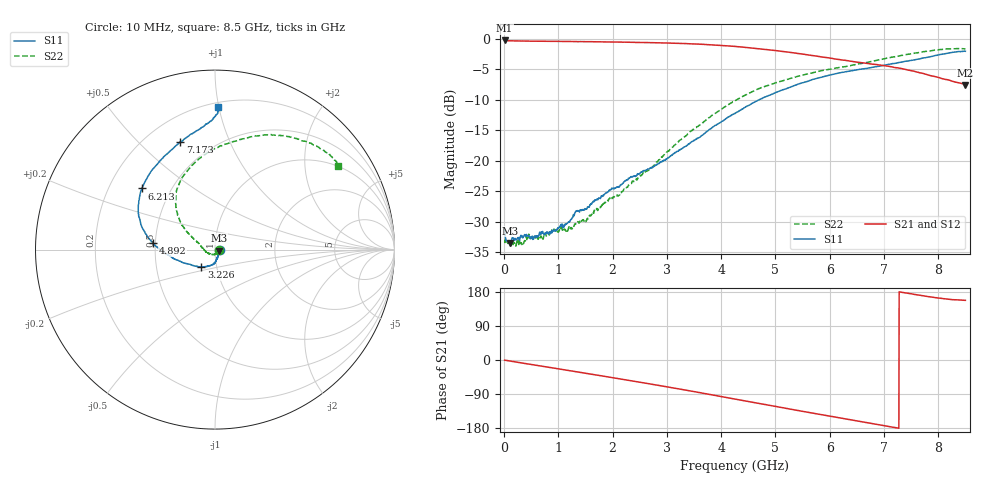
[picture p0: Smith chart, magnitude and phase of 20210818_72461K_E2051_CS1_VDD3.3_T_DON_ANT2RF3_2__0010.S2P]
!Agilent Technologies,E5071C,MY46417908,A.11.23
!Date: Wed Aug 18 14:29:43 2021
!Data & Calibration Information:
!Freq	S11:SOLT2(ON)	S21:SOLT2(ON)	S12:SOLT2(ON)	S22:SOLT2(ON)
!PortZ  Port1:50+j0  Port2:50+j0
!Above PortZ is port z conversion or system Z0 setting when saving the data.
!When reading, reference impedance value at option line is always used.
# Hz S dB R 50
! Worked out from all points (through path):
!   1601 points, 10 MHz to 8.5 GHz, reference 50 ohm
!   highest |S21| = -0.24 dB at 10 MHz (marker M1); lowest = -7.5 dB at 8.5 GHz (marker M2)
!   group delay of S21, straight-line fit = 69 ps
!   lowest |S11| = -33.5 dB at 110.8 MHz (marker M3), VSWR 1.04, Z = 52.1 - j0.533 ohm
!   |S11| at or under -10 dB: start of sweep to 4.69 GHz
!   |S22| runs from -34.0 to -1.6 dB; largest |S21 - S12| = 0.0047
!   S11 on the Smith chart (normalised r, x): 10 MHz: 1.05, +0.00; 3.226 GHz: 0.84, -0.17; 4.892 GHz: 0.49, +0.04; 6.213 GHz: 0.34, +0.32; 7.173 GHz: 0.34, +0.67; 8.5 GHz: 0.23, +1.00
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1e7  -31.69 0.7  -0.24 -0.4  -0.24 -0.4  -33.22 -8.8
1.108188e8  -33.48 -14.0  -0.29 -2.8  -0.29 -2.8  -33.65 -18.7
3.28375e8  -32.30 -25.3  -0.33 -7.8  -0.32 -7.8  -33.66 -45.1
4.451125e8  -32.23 -35.5  -0.34 -10.6  -0.33 -10.6  -32.46 -49.6
6.838938e8  -31.92 -44.8  -0.37 -16.0  -0.36 -16.0  -32.41 -62.0
8.483875e8  -31.86 -54.9  -0.39 -19.8  -0.39 -19.8  -32.00 -74.9
1.177375e9  -30.14 -59.7  -0.41 -27.4  -0.41 -27.4  -31.35 -95.8
1.320644e9  -28.33 -65.4  -0.42 -30.7  -0.42 -30.7  -30.27 -114.2
1.426769e9  -28.16 -67.3  -0.43 -33.2  -0.43 -33.2  -29.72 -125.1
1.516975e9  -27.90 -68.5  -0.44 -35.3  -0.44 -35.3  -29.76 -130.0
2.185562e9  -23.72 -86.7  -0.52 -51.1  -0.52 -51.1  -24.93 -173.9
2.843538e9  -20.41 -108.7  -0.62 -67.0  -0.63 -67.0  -19.93 158.3
3.225588e9  -18.21 -128.2  -0.72 -76.4  -0.72 -76.4  -16.71 151.8
3.692538e9  -15.51 -151.6  -0.88 -88.4  -0.88 -88.4  -13.50 144.7
4.255e9  -12.21 -170.1  -1.22 -103.0  -1.21 -103.0  -10.15 133.6
4.89175e9  -9.22 174.2  -1.79 -119.6  -1.79 -119.6  -7.52 118.0
5.671769e9  -6.69 156.3  -2.70 -139.8  -2.72 -140.0  -5.55 97.0
6.213006e9  -5.49 140.1  -3.41 -153.3  -3.41 -153.5  -4.61 85.2
7.088538e9  -4.16 110.4  -4.49 -175.6  -4.49 -175.7  -3.09 65.8
7.173438e9  -4.03 108.0  -4.64 -177.6  -4.63 -177.6  -2.94 64.0
7.916312e9  -2.78 91.0  -6.12 165.3  -6.09 165.2  -1.85 45.3
8.5e9  -2.01 88.7  -7.54 157.4  -7.45 157.5  -1.64 34.3
